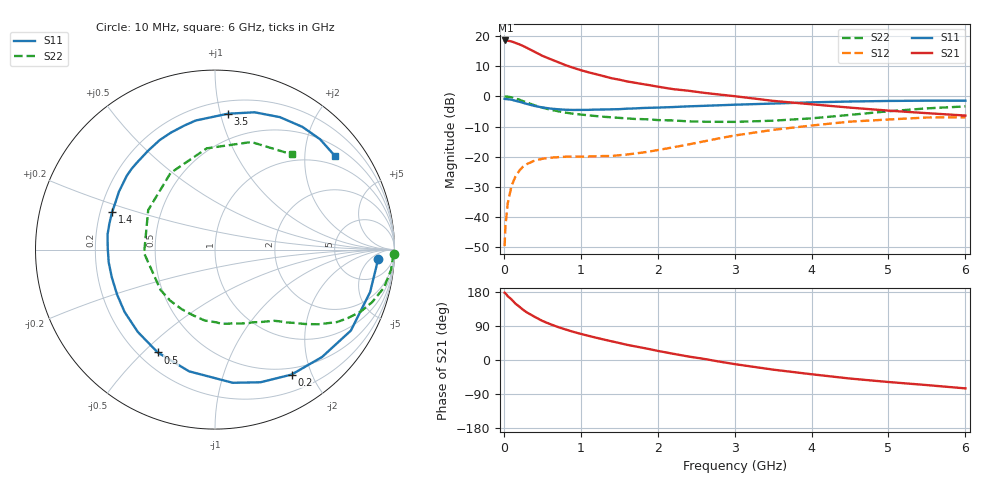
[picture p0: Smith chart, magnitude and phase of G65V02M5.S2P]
! SIEMENS Small Signal Semiconductors
! BFG193
! Si NPN RF Bipolar Junction Transistor in SOT223
! VCE = 5 V  IC = 2.5 mA
! Common Emitter S-Parameters:  August  1996
# GHz  S  MA  R  50
!  f  S11  S21  S12  S22
! GHz  MAG  ANG  MAG  ANG  MAG  ANG  MAG  ANG
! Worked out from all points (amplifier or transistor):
!   36 points, 10 MHz to 6 GHz, reference 50 ohm
!   highest |S21| = 18.5 dB at 20 MHz (marker M1)
!   |S21| within 3 dB of that: start of sweep to 341.9 MHz
!   unconditionally stable (mu >= 1): 1.32 GHz to 2.542 GHz
!   at 250 MHz: K = 0.21, MSG = 20.0 dB, |S12| = -23.3 dB
!   at 1.4 GHz: K = 1.06, MAG = 11.4 dB, |S12| = -19.8 dB
!   at 6 GHz: K = 0.93, MSG = 0.3 dB, |S12| = -6.9 dB
!   S11 on the Smith chart (normalised r, x): 10 MHz: 16, -9; 200 MHz: 0.41, -1.71; 500 MHz: 0.28, -0.55; 1.4 GHz: 0.25, +0.17; 3.5 GHz: 0.29, +1.06; 6 GHz: 0.73, +2.71
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0.01  0.91 -3.2  8.415 177.6  0.0033 91.7  0.9965 -1.3
0.02  0.9034 -6.3  8.435 176.4  0.0069 87.0  0.9921 -2.6
0.05  0.8961 -15.3  8.359 168.7  0.0168 80.6  0.9873 -6.6
0.1  0.8812 -30.8  8.126 159.8  0.033 73.9  0.965 -12.7
0.15  0.8448 -45.1  7.691 149.0  0.0467 65.2  0.923 -18.5
0.2  0.8166 -58.5  7.286 141.0  0.0585 59.2  0.8829 -23.0
0.25  0.7813 -71.1  6.844 132.6  0.0685 52.9  0.8326 -27.3
0.3  0.7486 -82.4  6.36 125.5  0.0756 48.4  0.7906 -30.7
0.4  0.6935 -102.0  5.471 114.0  0.0863 40.3  0.7113 -35.8
0.5  0.6558 -119.1  4.701 103.2  0.0923 34.2  0.6503 -39.6
0.6  0.6288 -133.1  4.168 94.9  0.0964 30.4  0.6037 -42.6
0.7  0.612 -145.4  3.707 87.3  0.0983 27.7  0.5688 -45.5
0.9  0.5953 -165.1  2.982 74.5  0.1009 24.4  0.5165 -50.2
1.1  0.5976 179.3  2.503 63.8  0.1009 24.1  0.4845 -56.1
1.4  0.6102 159.8  1.997 49.4  0.1029 26.4  0.4502 -65.3
1.7  0.6312 144.3  1.684 36.2  0.1128 30.8  0.4225 -76.1
2.2  0.6653 124.0  1.318 16.5  0.1431 34.3  0.3992 -98.3
2.8  0.7116 104.0  1.072 -4.2  0.2018 30.6  0.3785 -131.3
3.5  0.7604 84.6  0.842 -25.4  0.2787 16.4  0.3954 -177.1
4.5  0.8218 63.9  0.651 -48.9  0.3816 -6.9  0.4935 120.1
5.5  0.8489 46.4  0.527 -66.2  0.4467 -35.5  0.6328 71.3
6  0.8476 38.2  0.481 -74.9  0.4504 -50.9  0.6813 51.2
